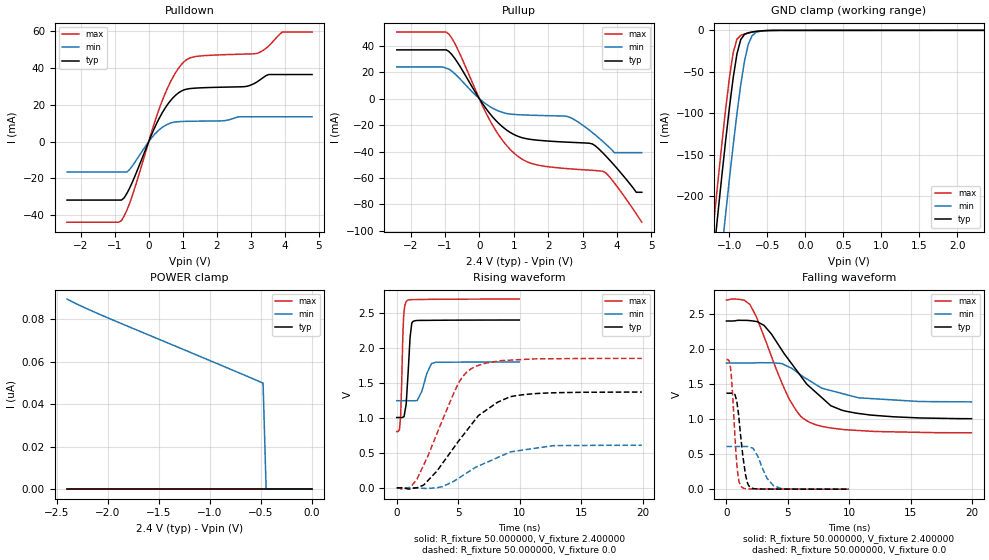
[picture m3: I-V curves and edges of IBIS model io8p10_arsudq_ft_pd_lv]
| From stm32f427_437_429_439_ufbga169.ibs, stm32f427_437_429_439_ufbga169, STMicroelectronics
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|   Model io8p10_arsudq_ft_pd_lv
[Model]  io8p10_arsudq_ft_pd_lv
Model_type I/O
Polarity   Non-Inverting
Enable   Active-Low
Vinl =   0.720000V
Vinh =   1.680000V
Vmeas =  1.200000V
Cref =   40.000000pF
Rref =   100.000000M
Vref =   0.0V
C_comp   2.239000pF   2.178700pF   2.334000pF
[Temperature Range]   25.000000   0.125000k   -40.000000
[Pullup Reference]   2.400000V   1.800000V   2.700000V
[Pulldown Reference]   0.0V   0.0V   0.0V
[POWER Clamp Reference]   2.400000V   1.800000V   2.700000V
[GND Clamp Reference]   0.0V   0.0V   0.0V
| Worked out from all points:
|   slope of the pulldown table from 0 to 0.36 V, typ, clamps not added: 25 ohm
|   slope of the pullup table from 0 to 0.36 V, typ, clamps not added: 27.7 ohm
|   GND clamp passes 1 mA (typ) near -0.62 V on its own axis
|   rising waveform, R_fixture 50.000000, V_fixture 2.400000: 20-80 % time 277ps typ, 617ps min, 183ps max; typ from 1 V to 2.4 V
|   rising waveform, R_fixture 50.000000, V_fixture 0.0: 20-80 % time 3.74ns typ, 4.02ns min, 2.67ns max; typ from 0 V to 1.37 V
|   falling waveform, R_fixture 50.000000, V_fixture 2.400000: 20-80 % time 3.89ns typ, 4ns min, 2.72ns max; typ from 2.4 V to 1 V
|   falling waveform, R_fixture 50.000000, V_fixture 0.0: 20-80 % time 528ps typ, 976ps min, 382ps max; typ from 1.37 V to 0 V
[Pulldown]
|Voltage   I(typ)   I(min)   I(max)
-2.4V     -31.73mA   -16.51mA   -43.74mA
-800mV    -31.73mA   -16.51mA   -42.87mA
-480mV    -21.98mA   -13.17mA   -29.2mA
80mV      3.63mA     1.966mA    5.014mA
480mV     18.15mA    8.738mA    26.02mA
800mV     25.38mA    10.72mA    37.77mA
1.12V     28.53mA    11.02mA    44.6mA
2.8V      29.84mA    13.49mA    47.53mA
3.2V      32.65mA    13.49mA    48.04mA
3.52V     36.42mA    13.49mA    51.83mA
3.92V     36.42mA    13.49mA    59.49mA
4.8V      36.42mA    13.49mA    59.49mA
[Pullup]
|Voltage   I(typ)   I(min)   I(max)
-2.4V     36.91mA    24.03mA    50.37mA
-960mV    36.91mA    23.05mA    50.37mA
-640mV    27.65mA    17.03mA    37.99mA
320mV     -11.75mA   -6.207mA   -17.08mA
960mV     -26.47mA   -11.82mA   -40.02mA
1.52V     -30.88mA   -12.51mA   -49.05mA
2.56V     -32.88mA   -13.48mA   -52.9mA
3.28V     -34.19mA   -25.52mA   -54.18mA
3.6V      -41.31mA   -32.62mA   -54.97mA
3.92V     -50.32mA   -40.8mA    -63.63mA
4.56V     -70.8mA    -40.8mA    -87.08mA
4.72V     -70.8mA    -40.8mA    -93.4mA
[GND_clamp]
|Voltage   I(typ)   I(min)   I(max)
-2.4V     -1.424A    -1.508A    -1.393A
-1.25V    -311.2mA   -401.9mA   -273.3mA
-1.2V     -265.4mA   -356.1mA   -227.2mA
-1.15V    -220.4mA   -310.8mA   -181.9mA
-1.1V     -176.3mA   -266.2mA   -137.9mA
-1.05V    -133.8mA   -222.5mA   -95.87mA
-950mV    -57.3mA    -138.9mA   -26.99mA
-900mV    -28.28mA   -100.4mA   -10.6mA
-850mV    -11.02mA   -65.54mA   -5.972mA
-750mV    -2.846mA   -16.51mA   -3.192mA
-600mV    -761.3uA   -1.173mA   -751.9uA
2.35V     58.09uA    37.92uA    67.25uA
[POWER_clamp]
|Voltage   I(typ)   I(min)   I(max)
-2.4V     0A         89.62nA    0A
-2.04V    0A         81.57nA    0A
-480mV    0A         50.01nA    0A
-450mV    0A         0A         0A
0V        0A         0A         0A
[Ramp]
| variable   typ   min   max
dV/dt_r  0.82146/3.73951n   0.36560/4.02298n   1.11330/2.67421n
dV/dt_f  0.83346/3.89472n   0.33288/4.07556n   1.13629/2.72402n
R_load = 50.000000
[Rising Waveform]
R_fixture= 50.000000
V_fixture= 2.400000
V_fixture_min= 1.800000
V_fixture_max= 2.700000
|time   V(typ)   V(min)   V(max)
0s        1.005V     1.245V     804.2mV
220.2ps   1.005V     1.245V     830.8mV
300.3ps   1.005V     1.245V     989.3mV
560.6ps   1.014V     1.246V     2.438V
820.8ps   1.346V     1.246V     2.673V
1.081ns   2.138V     1.245V     2.689V
1.341ns   2.38V      1.244V     2.69V
2.042ns   2.393V     1.379V     2.693V
2.843ns   2.395V     1.777V     2.695V
9.97ns    2.399V     1.799V     2.698V
[Rising Waveform]
R_fixture= 50.000000
V_fixture= 0.0
V_fixture_min= 0.0
V_fixture_max= 0.0
|time   V(typ)   V(min)   V(max)
0s        168.8uV    66.4uV     586uV
1.121ns   -14.77mV   125.1uV    12.42mV
1.642ns   539.4uV    -516.2uV   122.2mV
3.283ns   242.6mV    2.475mV    780mV
5.005ns   662.7mV    134.6mV    1.49V
6.206ns   934.1mV    271.2mV    1.717V
8.168ns   1.22V      429.5mV    1.809V
9.57ns    1.313V     522.2mV    1.829V
12.77ns   1.358V     603.5mV    1.846V
19.94ns   1.369V     608.4mV    1.85V
[Falling Waveform]
R_fixture= 50.000000
V_fixture= 2.400000
V_fixture_min= 1.800000
V_fixture_max= 2.700000
|time   V(typ)   V(min)   V(max)
0s        2.399V     1.799V     2.698V
1.441ns   2.408V     1.799V     2.696V
1.922ns   2.404V     1.8V       2.631V
3.043ns   2.339V     1.804V     2.184V
5.085ns   1.842V     1.743V     1.291V
6.006ns   1.624V     1.635V     1.047V
6.727ns   1.468V     1.552V     957.7mV
8.488ns   1.191V     1.407V     872.9mV
9.77ns    1.11V      1.348V     847mV
19.94ns   1.005V     1.245V     804.2mV
[Falling Waveform]
R_fixture= 50.000000
V_fixture= 0.0
V_fixture_min= 0.0
V_fixture_max= 0.0
|time   V(typ)   V(min)   V(max)
0s        1.369V     608.4mV    1.85V
340.3ps   1.369V     608.4mV    1.719V
440.4ps   1.369V     608.4mV    1.521V
700.7ps   1.345V     608.3mV    727mV
940.9ps   1.126V     608.1mV    197mV
1.241ns   623.6mV    607.9mV    30.66mV
1.682ns   104.4mV    609.6mV    4.924mV
2.042ns   16.68mV    590.8mV    2.861mV
3.844ns   1.254mV    48.1mV     1.416mV
9.97ns    168.8uV    66.4uV     586uV
